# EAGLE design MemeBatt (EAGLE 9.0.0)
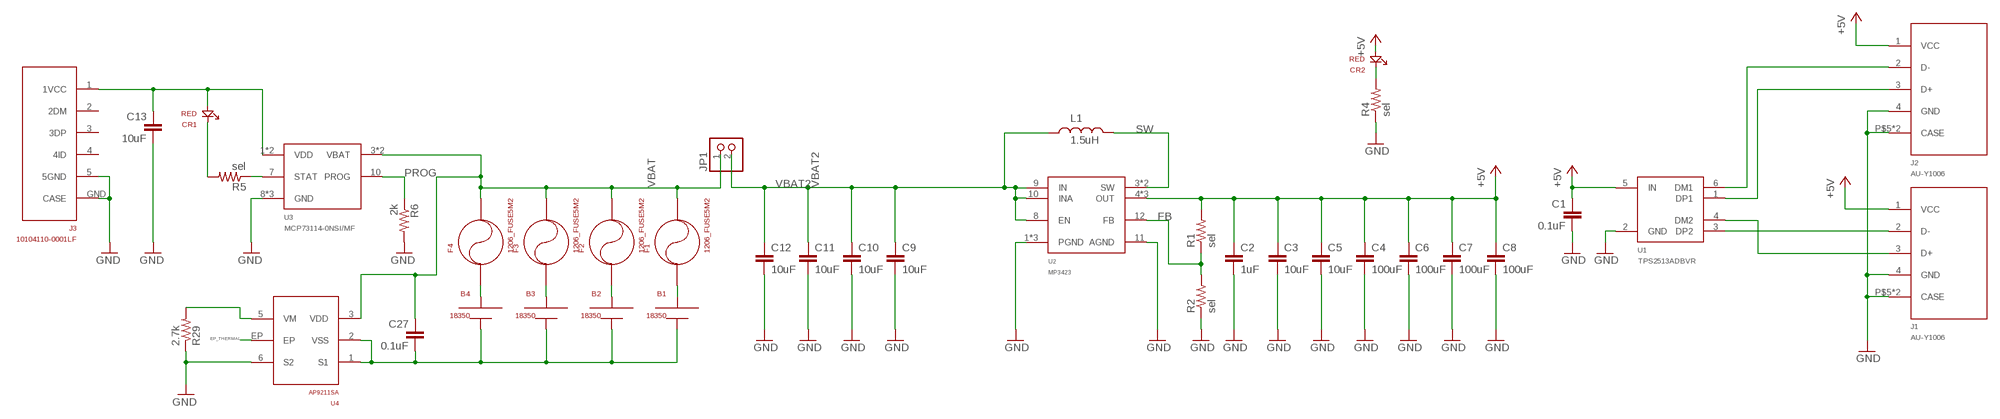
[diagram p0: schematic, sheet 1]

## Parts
B1  18350  [18350]
B2  18350  [18350]
B3  18350  [18350]
B4  18350  [18350]
C1  0.1uF  0603_CAPACITOR  [0603]
C2  1uF  0603_CAPACITOR  [0603]
C3  10uF  0805_CAPACITOR  [0805]
C4  100uF  1210_CAPACITOR  [1210]
C5  10uF  0805_CAPACITOR  [0805]
C6  100uF  1210_CAPACITOR  [1210]
C7  100uF  1210_CAPACITOR  [1210]
C8  100uF  1210_CAPACITOR  [1210]
C9  10uF  0805_CAPACITOR  [0805]
C10  10uF  0805_CAPACITOR  [0805]
C11  10uF  0805_CAPACITOR  [0805]
C12  10uF  0805_CAPACITOR  [0805]
C13  10uF  0805_CAPACITOR  [0805]
C27  0.1uF  0603_CAPACITOR  [0603]
CR1  RED  150060RS75000  [0603_DIODE]
CR2  RED  150060RS75000  [0603_DIODE]
F1  1206_FUSE5M2  [1206_FUSE_5M2]
F2  1206_FUSE5M2  [1206_FUSE_5M2]
F3  1206_FUSE5M2  [1206_FUSE_5M2]
F4  1206_FUSE5M2  [1206_FUSE_5M2]
J1  AU-Y1006  [USBA_SMD]
J2  AU-Y1006  [USBA_SMD]
J3  10104110-0001LF  [MICRO_USB]
JP1  PINHD-1X2  [1X02]
L1  1.5uH  NRS8030T1R5NJGJ  [NRS8030]
R1  sel  0603_RESISTOR  [0603]
R2  sel  0603_RESISTOR  [0603]
R4  sel  0603_RESISTOR  [0603]
R5  sel  0603_RESISTOR  [0603]
R6  2k  0603_RESISTOR  [0603]
R29  2.7k  0603_RESISTOR  [0603]
U1  TPS2513ADBVR  [SOT23-6]
U2  MP3423  [QFN14_MPS]
U3  MCP73114-0NSI/MF  [10DFN]
U4  AP9211SA  [AP9211SA]

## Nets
+5V: C1.1 C2.1 C3.1 C4.1 C5.1 C6.1 C7.1 C8.1 CR2.A J1.1(VCC) J2.1(VCC) R1.2 U1.5(IN) U2.4(OUT) U2.5(OUT) U2.6(OUT)
BAT-: B1.- B2.- B3.- B4.- C27.2 U4.1(S1) U4.2(VSS)
EP_THERMAL: U4.EP
FB: R1.1 R2.2 U2.12(FB)
GND: C1.2 C2.2 C3.2 C4.2 C5.2 C6.2 C7.2 C8.2 C9.2 C10.2 C11.2 C12.2 C13.2 J1.4(GND) J1.P$5(CASE) J1.P$6(CASE) J2.4(GND) J2.P$5(CASE) J2.P$6(CASE) J3.5(5GND) J3.GND(CASE) R2.1 R4.1 R6.2 R29.1 U1.2(GND) U2.1(PGND) U2.2(PGND) U2.11(AGND) U2.13(PGND) U3.8(GND) U3.9(GND) U3.GF(GND) U4.6(S2)
N$2: B1.+ F1.P$1
N$3: B4.+ F4.P$1
N$4: B3.+ F3.P$1
N$5: J2.2(D-) U1.6(DM1)
N$6: J2.3(D+) U1.1(DP1)
N$7: J1.3(D+) U1.4(DM2)
N$8: J1.2(D-) U1.3(DP2)
N$9: B2.+ F2.P$1
N$10: CR2.K R4.2
N$13: CR1.K R5.2
N$24: R29.2 U4.5(VM)
PROG: R6.1 U3.10(PROG)
STAT: R5.1 U3.7(STAT)
SW: L1.P$2 U2.3(SW) U2.14(SW)
VBAT: C27.1 F1.P$2 F2.P$2 F3.P$2 F4.P$2 JP1.1 U3.3(VBAT) U3.4(VBAT) U4.3(VDD)
VBAT2: C9.1 C10.1 C11.1 C12.1 JP1.2 L1.P$1 U2.8(EN) U2.9(IN) U2.10(INA)
VIN: C13.1 CR1.A J3.1(1VCC) U3.1(VDD) U3.2(VDD)
Unconnected: J3.2(2DM) J3.3(3DP) J3.4(4ID)

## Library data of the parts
B1-B4 = ruark2:18350: Ecigarette Battery
C1 C2 C27 = ruark2:0603_CAPACITOR: 0603 Capacitor -- WARNING: NO DEFINED VALUE OR PART NUMBER; VALUE: sel
C3 C5 C9-C13 = ruark2:0805_CAPACITOR: NO DEFINED PN
C4 C6-C8 = ruark2:1210_CAPACITOR: NO VALUE
CR1 CR2 = ruark2:150060RS75000: Red 625nm LED Indication - Discrete 2V 0603 (1608 Metric); PARTNO: 732-4978-1-ND
F1-F4 = ruark2:1206_FUSE
J1 J2 = ruark2:AU-Y1006: USB - A USB 1.1 Receptacle Connector 4 Position Surface Mount, Right Angle; PARTNO: AE11182-ND
J3 = ruark2:10104110-0001LF: USB - micro B USB 2.0 Receptacle Connector 5 Position Surface Mount, Right Angle; PARTNO: 609-4052-1-ND
JP1 = pinhead:PINHD-1X2: PIN HEADER
L1 = ruark2:NRS8030T1R5NJGJ: 1.5 µH Shielded Drum Core, Wirewound Inductor 5.3 A 15.6mOhm Max Nonstandard; PARTNO: 587-2963-1-ND
R1 R2 R4 R5 = ruark2:0603_RESISTOR: 0603 Resistor -- WARNING: NO DEFINED PART NUMBER OR VALUE
R6 R29 = ruark2:0603_RESISTOR: 0603 Resistor -- WARNING: NO DEFINED PART NUMBER OR VALUE; VALUE: sel
U1 = ruark2:TPS2513ADBVR: USB Dedicated Charging Port (DCP), Power Switch PMIC SOT-23-6
U2 = ruark2:MP3423: Boost Switching Regulator IC Positive Adjustable 2.5V 1 Output 9A (Switch) 14-PowerVFQFN; PARTNO: 1589-1171-1-ND
U3 = ruark2:MCP73114-0NSI/MF: Charger IC Lithium Ion/Polymer 10-DFN (3x3); PARTNO: MCP73114-0NSI/MF-ND
U4 = ruark2:AP9211SA: Battery Battery Protection IC Lithium-Ion U-DFN2030-6 (Type C); PARTNO: AP9211SA-AE-HAC-7DICT-ND

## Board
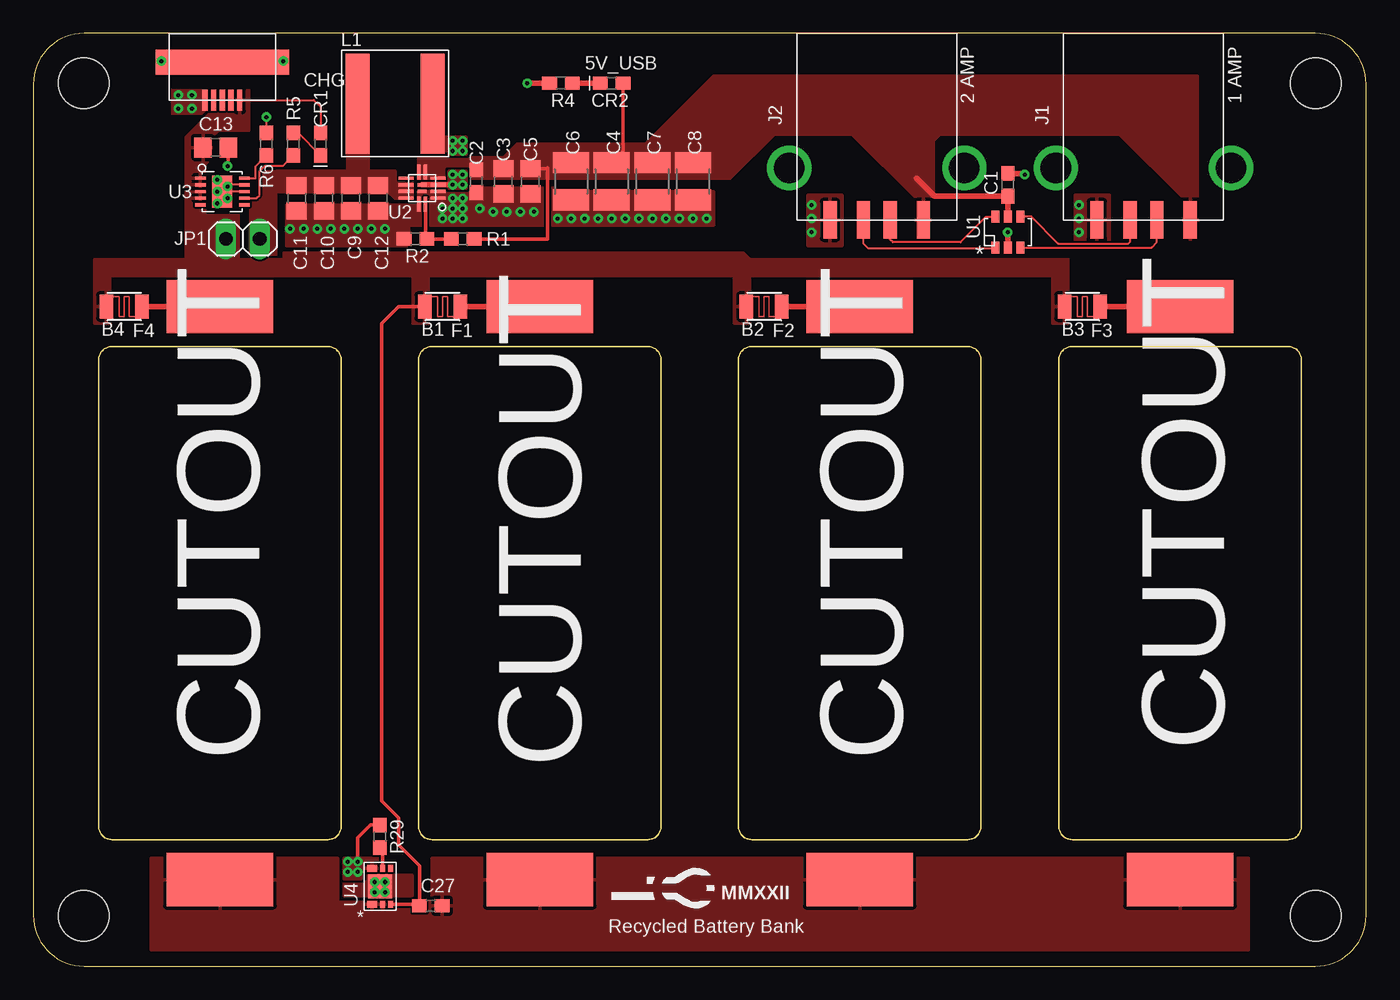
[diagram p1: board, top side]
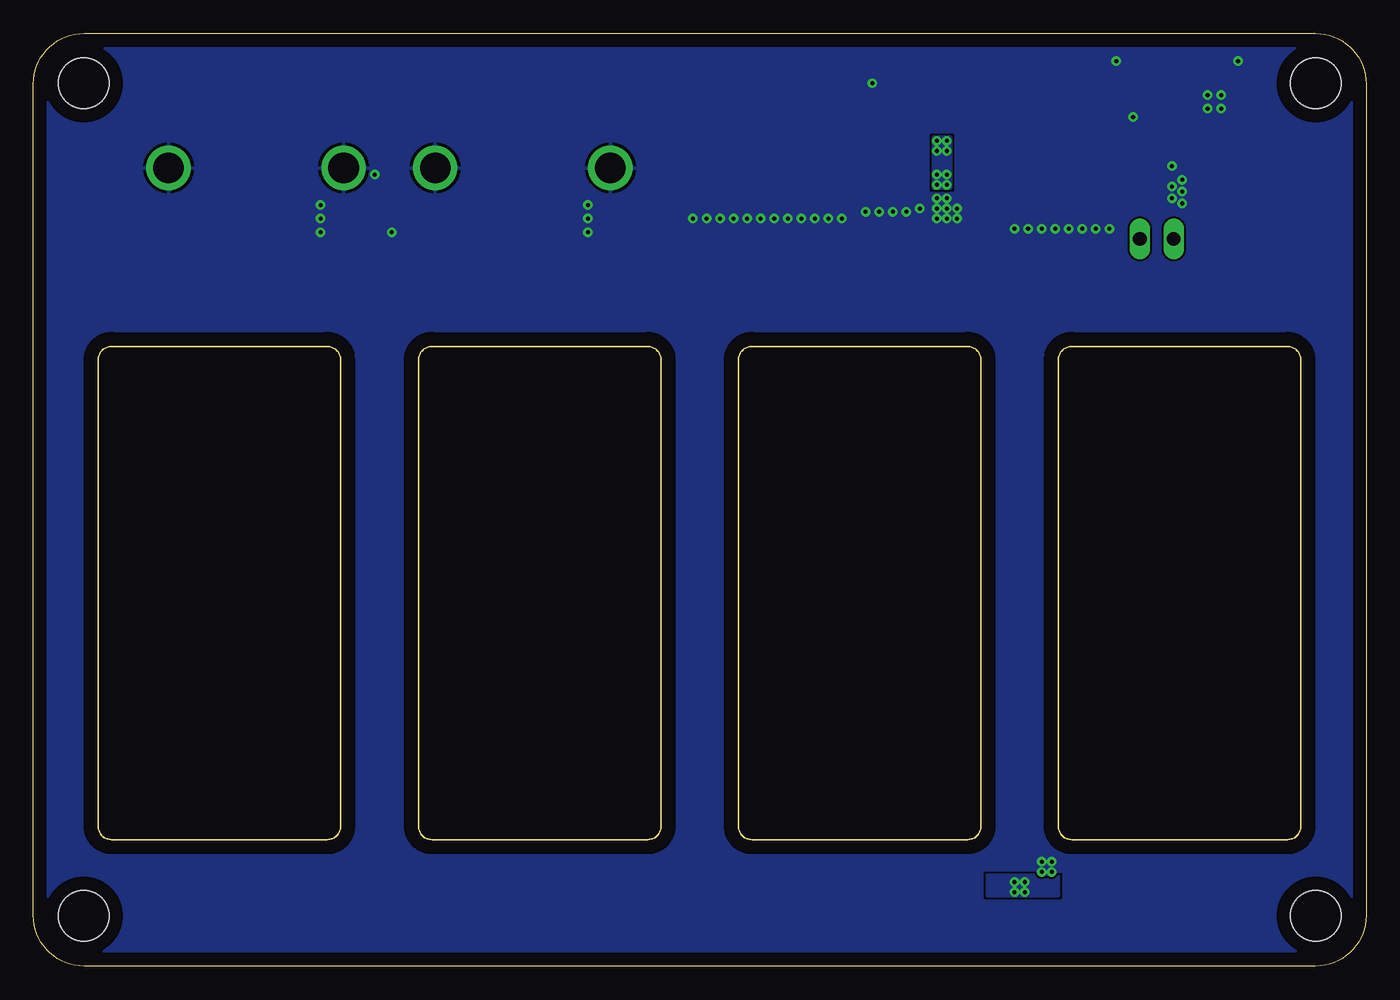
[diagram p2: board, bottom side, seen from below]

Size 100 x 70 mm. Coordinates in mm from the lower left corner, seen from the top.
Outline: 0,66.19 0,3.81 arc90 3.81,0 96.19,0 arc90 100,3.81 100,66.19 arc90 96.19,70 3.81,70 arc90 0,66.19
Copper layers (1*16): Top 0.035mm / dielectric 1.5mm / Bottom 0.035mm
Design rules "default *": minimum track width 5mil, minimum drill 12mil, track to track 6mil, track to pad 6mil, pad to pad 6mil, via to via 6mil, smd to smd 6mil, copper to edge 40mil, drill to drill 6mil, minimum pad ring 10mil, minimum via ring 8mil, stop-mask expansion 4mil, vias tented up to drill 12mil, thermal gap 10mil
Holes 3.81 mm at 3.77,3.77 96.23,3.77 3.77,66.26 96.23,66.26

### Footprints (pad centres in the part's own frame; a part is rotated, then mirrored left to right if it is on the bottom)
18350 = smd 8 x 4: + 0,21.5; - 0,-21.5
0603 = smd 1.1 x 1: 1 -0.85,0; 2 0.85,0
0805 = smd 1.3 x 1.5: 1 -0.95,0; 2 0.95,0
1210 = smd 1.6 x 2.7: 1 -1.4,0; 2 1.4,0
0603_DIODE = smd 1.1 x 1: A -0.85,0; K 0.85,0
1206_FUSE_5M2 = smd 1.016 x 1.778: P$1 -1.333,0; P$2 1.333,0
USBA_SMD = smd 1 x 2.8: 1 -3.5,0; 2 -1,0; 3 1,0; 4 3.5,0 | drill 2.3: P$5 6.57,-3.9; P$6 -6.57,-3.9
MICRO_USB = smd 0.4 x 1.6: 1 -1.3,0; 2 -0.65,0; 3 0,0; 4 0.65,0; 5 1.3,0 | smd 10 x 1.9: GND 0,-2.84
1X02 = drill 1.016 long: 1 -1.27,0; 2 1.27,0
NRS8030 = smd 1.8 x 7.5: P$1 -2.8,0; P$2 2.8,0
SOT23-6 = smd 0.6 x 0.9: 1 -0.95,-1.15; 2 0,-1.15; 3 0.95,-1.15; 4 0.95,1.15; 5 0,1.15; 6 -0.95,1.15
QFN14_MPS = smd 1.1 x 0.25: 1 -1.2,0.75; 2 -1.2,0.25; 3 -1.2,-0.25; 4 -1.2,-0.75; 7 1.2,-0.75; 8 1.2,-0.25; 9 1.2,0.25; 10 1.2,0.75 | smd 0.25 x 1.1: 5 -0.25,-1.2; 6 0.25,-1.2; 11 0.25,1.2; 12 -0.25,1.2 | smd 0.7 x 0.25: 13 0,0.25; 14 0,-0.25
10DFN = smd 0.8 x 0.24: 1 -1.65,1; 2 -1.65,0.5; 3 -1.65,0; 4 -1.65,-0.5; 5 -1.65,-1; 6 1.65,-1; 7 1.65,-0.5; 8 1.65,0; 9 1.65,0.5; 10 1.65,1 | smd 1.5 x 2.4: GF 0,0
AP9211SA = smd 0.75 x 0.5: 1 -0.575,-1.35; 6 -0.575,1.35 | smd 0.4 x 0.5: 2 0.2,-1.35; 3 0.8,-1.35; 4 0.8,1.35; 5 0.2,1.35 | smd 1.8 x 1.8: EP 0,0

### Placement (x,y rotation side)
B1  38,28 0 top
B2  62,28 0 top
B3  86.04,28 0 top
B4  14,28 0 top
C1  73.11,58.64 90 top
C2  33.24,58.89 270 top
C3  35.27,58.89 270 top
C4  43.4,58.89 270 top
C5  37.3,58.89 270 top
C6  40.35,58.89 270 top
C7  46.44,58.89 270 top
C8  49.49,58.89 270 top
C9  23.84,57.62 270 top
C10  21.81,57.62 270 top
C11  19.77,57.62 270 top
C12  25.87,57.62 270 top
C13  13.68,61.43 0 top
C27  29.82,4.53 0 top
CR1  21.55,61.68 270 top
CR2  43.4,66.26 180 top
F1  30.7,49.49 180 top
F2  54.83,49.49 180 top
F3  78.7,49.49 180 top
F4  6.82,49.49 180 top
J1  83.29,56 180 top
J2  63.28,56 180 top
J3  14.19,64.99 180 top
JP1  15.71,54.57 0 top
L1  27.14,64.73 0 top
R1  32.22,54.57 0 top
R2  28.66,54.57 0 top
R4  39.59,66.26 0 top
R5  19.52,61.68 90 top
R6  17.49,61.68 90 top
R29  26,9.74 270 top
U1  73.11,55.08 0 top
U2  29.17,58.38 180 top
U3  14.19,58.13 0 top
U4  26,6 0 top

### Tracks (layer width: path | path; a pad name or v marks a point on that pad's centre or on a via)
+5V
  Top 0.254: R1.2 38.57,54.57 38.57,59.84 | 38.57,59.91 38.57,59.84 | 38.57,59.84 C5.1 | CR2.A 44.25,61.14 C4.1
  Top 0.406: U1.5 C1.1 67.61,57.79 66.26,59.14
  pour Top (rank 2, no thermals): 28.92,59.14 51.02,59.14 51.02,61.68 36.28,61.68 35.27,60.67 28.92,60.67
  pour Top: 43.4,59.14 52.29,59.14 55.59,62.45 61.43,62.45 66.26,57.62 66.26,54.57 67.27,54.57 67.27,57.62 67.53,57.87 67.53,61.94 68.03,62.45 81.5,62.45 86.32,57.62 86.32,54.57 87.34,54.57 87.34,66.76 51.02,66.76
BAT-
  pour Top: 8.85,8.09 22.82,8.09 22.82,4.79 29.93,4.79 29.93,8.09 91.15,8.09 91.15,1.23 8.85,1.23
EP_THERMAL  (via drill 0.3)
  other vias: 26.38,6.31 25.62,6.31 25.62,5.55 26.38,5.55
  pour Bottom: 23.08,5.3 28.41,5.3 28.41,6.82 23.08,6.82
  pour Top (rank 3, no thermals): 23.33,5.3 28.41,5.3 28.41,6.82 25.11,6.82 25.11,6.31 23.33,6.31
FB
  Top 0.254: U2.12 29.42,54.57 R2.2 R1.1
GND  (via drill 0.3)
  Top 0.152: U3.GF v13.8,58.13 | U3.9 14.69,58.63 v14.57,58.51 14.95,58.13 U3.8 | R6.2 v17.49,63.72 | J3.GND 18.68,67.83 v18.76,67.91
  Top 0.254: C13.2 14.63,60.09 v14.57,60.03 | R29.1 25.32,10.59 24.35,9.61 v24.35,7.84
  Top 0.406: U1.2 v73.11,55.08 | C1.2 74.3,59.49 v74.38,59.4 | R4.1 v37.05,66.26
  other vias: 31.46,57.62 32.22,57.62 32.22,56.86 31.46,56.86 30.7,56.86 30.7,56.1 31.46,56.1 32.22,56.1 33.49,56.86 34.51,56.6 35.52,56.6 36.54,56.6 37.55,56.6 40.35,56.1 39.33,56.1 41.36,56.1 43.4,56.1 42.38,56.1 44.41,56.1 45.43,56.1 46.44,56.1 47.46,56.1 48.48,56.1 49.49,56.1 50.51,56.1 26.38,55.33 25.36,55.33 24.35,55.33 23.33,55.33 22.31,55.33 21.3,55.33 20.28,55.33 19.27,55.33 58.38,57.11 58.38,56.1 58.38,55.08 78.45,56.1 78.45,57.11 78.45,55.08 13.8,57.24 14.57,57.62 13.8,59.02 11.9,65.37 11.9,64.35 10.88,64.35 10.88,65.37 9.61,67.91 23.58,7.84 23.58,7.07 24.35,7.07
  pour Bottom (rank 2): 0.22,70.07 96.23,70.07 arc-90 100.04,66.26 100.04,-0.04 -0.04,-0.04 -0.04,70.07
  pour Top (rank 2, no thermals): 19.01,57.11 28.92,57.11 28.92,58.13 32.98,58.13 32.98,58.38 39.08,58.38 39.08,58.13 51.02,58.13 51.02,55.59 28.16,55.59 28.16,54.32 arc-90 27.9,54.06 19.01,54.06
  pour Top (no thermals): 12.92,64.22 12.92,65.75 10.38,65.75 10.38,63.97 12.41,63.97 12.66,63.97
  pour Top: 25.87,7.07 24.6,7.07 24.6,6.57 23.33,6.57 23.33,8.09 25.87,8.09
  pour Top: 58.13,57.87 58.13,54.06 60.67,54.06 60.67,57.87
  pour Top: 78.19,57.87 78.19,54.06 80.73,54.06 80.73,57.87
N$2
  Top 0.406: F1.P$1 B1.+
N$3
  Top 0.406: F4.P$1 B4.+
N$4
  Top 0.406: F3.P$1 86.32,49.49 86.33,49.5 | 86.58,49.75 86.33,49.5 | 86.33,49.5 B3.+
N$5
  Top 0.152: U1.6 71.47,56.23 69.56,54.32 64.48,54.32 64.28,54.52 J2.2
N$6
  Top 0.152: U1.1 72.08,53.85 62.66,53.85 62.28,54.23 J2.3
N$7
  Top 0.152: 74.91,56.23 74.89,56.23 | 74.89,56.23 U1.4 | 74.89,56.23 76.89,54.23 82.17,54.23 82.29,54.35 J1.3
N$8
  Top 0.152: J1.2 84.29,54.32 83.9,53.93 U1.3
N$9
  Top 0.406: F2.P$1 B2.+
N$10
  Top 0.406: CR2.K R4.2
N$13
  Top 0.152: CR1.K 19.85,62.53 R5.2
N$24
  Top 0.254: U4.5 26.2,8.89 R29.2
PROG
  Top 0.152: U3.10 16.66,59.13 16.67,59.14 16.67,60.02 R6.1
STAT
  Top 0.152: U3.7 16.73,57.63 16.98,57.87 16.98,59.65 17.38,60.05 18.74,60.05 R5.1
SW  (via drill 0.3)
  Top 0.406: U2.14 31.2,58.64 | 31.2,58.64 v31.46,58.64 | U2.3 31.2,58.64
  other vias: 32.22,58.64 31.46,59.4 32.22,59.4 31.46,61.18 32.22,61.18 32.22,61.94 31.46,61.94
  pour Top (no thermals): 31.2,59.65 32.47,59.65 32.47,58.38 31.2,58.38
  pour Bottom: 31.2,58.38 32.47,58.38 32.47,62.19 31.2,62.19
  pour Top (no thermals): 29.17,61.18 31.2,61.18 31.2,60.92 32.47,60.92 32.47,62.19 30.7,62.19 30.7,68.29 29.17,68.29
VBAT
  Top 0.254: U4.3 28.97,4.65 | 28.97,4.65 C27.1 | F1.P$2 27.39,49.49 26.12,48.22 26.12,12.41 27.39,11.14 27.39,9.11 28.97,7.53 28.97,4.65
  pour Top: 18.76,53.05 15.46,53.05 15.46,56.35 12.92,56.35 12.92,58.13 11.39,58.13 11.39,53.05 4.53,53.05 4.53,48.22 5.8,48.22 5.8,51.78 28.41,51.78 28.41,48.22 29.68,48.22 29.68,51.78 52.54,51.78 52.54,48.22 53.81,48.22 53.81,51.78 76.42,51.78 76.42,48.22 77.69,48.22 77.69,53.05 53.81,53.05 53.3,53.56 18.76,53.56
  pour Top (no thermals): 15.46,52.54 15.46,56.35 12.92,56.35 12.92,52.54
VBAT2
  pour Top (no thermals): 18.25,58.13 26.63,58.13 27.14,57.62 28.41,57.62 28.41,58.89 27.14,58.89 27.14,59.65 25.11,59.65 25.11,68.29 23.58,68.29 23.58,59.65 18.25,59.65
  pour Top (rank 2, no thermals): 16.22,53.3 18.25,53.3 18.25,58.13 20.28,58.13 20.28,59.65 16.22,59.65
VIN
  Top 0.152: J3.1 21.04,64.99 21.55,64.48 CR1.A
  pour Top: 13.42,60.67 13.42,62.19 13.93,62.7 16.22,62.7 16.22,65.75 15.2,65.75 15.2,63.97 13.17,63.97 11.39,62.19 11.39,58.51 12.92,58.51 12.92,60.16

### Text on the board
tPlace: 5V_USB | CHG | 2 AMP | 1 AMP | CUTOUT | CUTOUT | CUTOUT | CUTOUT | MMXXII | Recycled Battery Bank
tStop: 023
